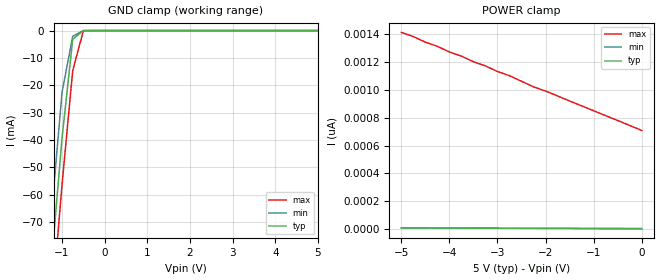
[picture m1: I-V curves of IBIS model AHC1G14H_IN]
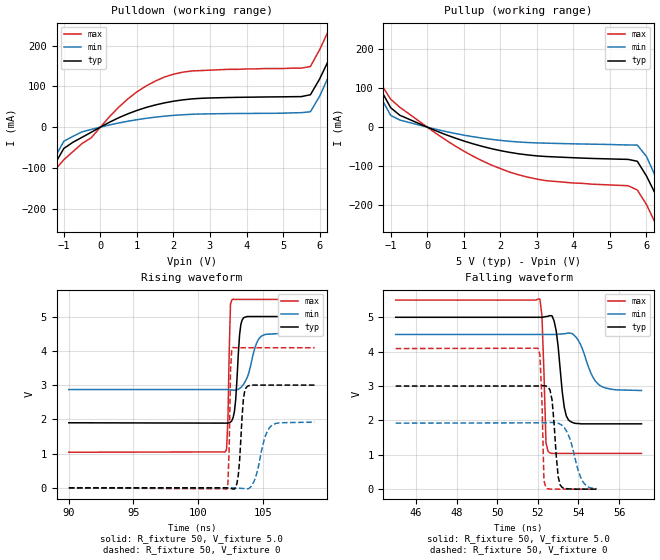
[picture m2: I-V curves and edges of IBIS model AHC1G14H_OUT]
| TEXAS INSTRUMENTS INCORPORATED
| Standard Linear and Logic Group
| IBIS Model of SN74AHC1G14H
| SINGLE SCHMITT-TRIGGER INVERTER
| CMPAK-5 5-pin (DCK) Package
[IBIS Ver]   2.1
[Comment Char]  |_char
[File name]   ul14_5c.ibs
[File Rev]   2.0
[Date]   April 17, 2000
[Source]   Data created from SPICE simulations at Hitachi,Ltd.
[Notes]   The following is an IBIS List for the AHC1G14H.
|   Please contact sllibis@ti.com with questions and
|   comments concerning SLL IBIS models.
[Disclaimer] Property of Texas Instruments Incorporated.  Unauthorized
   reproduction and/or distribution is strictly prohibited.
   This product is protected under copyright law.
   Created 2000, (C) Copyright 2000, Texas Instruments Inc.,
   All Rights Reserved.
   UNLESS THERE IS A SIGNED, WRITTEN AGREEMENT TO THE
   CONTRARY, TEXAS INSTRUMENTS () IS PROVIDING THE IBIS
   MODELS  AND WITHOUT ANY WARRANTY, EXPRESSED OR
   IMPLIED.  TI assumes no liability for:
   1) the accuracy of the IBIS models provided to your
   company;
   2) the proper functioning of these IBIS Models in your
   design or for any resulting applications; or
   3) infringement of patents, copyrights or intellectual
   property rights resulting from your use of these IBIS
   models.
   TI provides IBIS Models as a service to our customers.
   You and your company shall not distribute, sell or give
   these models to anyone else without prior written
   permission from TI.
   TI reserves the right to make changes to our products or
   to discontinue any semiconductor product or service
   without notice, and advises our customers to obtain the
   latest version of relevant information to verify, before
   placing orders, that the information being relied on is
   current.
   Please be aware that your receipt and use of the IBIS
   information provided shall serve as acceptance of these
   terms and conditions.  If you do not accept these terms,
   you should return or destroy the IBIS models and any
   other accompanying information immediately.
|   Component AHC1G14H
[Component]   AHC1G14H
[Manufacturer]   Hitachi, Ltd.
[Package]
|   typ   min   max
R_pkg   0.090   0.051   0.105
L_pkg   1.500nH   0.940nH   1.700nH
C_pkg   0.170pF   0.110pF   0.360pF
[Pin]   signal_name   model_name   R_pin   L_pin   C_pin
1   NC   NC   0.098   1.590nH   0.110pF
2   A   AHC1G14H_IN   0.051   0.940nH   0.170pF
3   GND   GND   0.092   1.590nH   0.360pF
4   Y   AHC1G14H_OUT   0.105   1.700nH   0.110pF
5   VCC   POWER   0.104   1.690nH   0.110pF
| Models and submodels in the file (2): AHC1G14H_IN (Input), AHC1G14H_OUT (Output)
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|   Model AHC1G14H_IN
[Model]   AHC1G14H_IN
Model_type  Input
Polarity   Non-Inverting
Vinl = 1.50
Vinh = 3.50
| variable   typ   min   max
C_comp   2.19pF   2.07pF   2.30pF
[Temperature Range]   25   85   -40
[Voltage Range]   5.0   4.5   5.5
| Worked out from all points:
|   GND clamp passes 1 mA (typ) near -0.58 V on its own axis
[GND Clamp]
|   Voltage   I(typ)   I(min)   I(max)
-5V       -823mA     -807mA     -840mA
-1.5V     -133mA     -115mA     -150mA
-1.25V    -85.2mA    -67.5mA    -103mA
-1V       -39.2mA    -22.5mA    -56.2mA
-750mV    -3.18mA    -2.09mA    -14.6mA
-500mV    -11.6uA    -2.99uA    -57.1uA
5V        5.34pA     5pA        708pA
[POWER Clamp]
|   Voltage   I(typ)   I(min)   I(max)
-5V       10.6pA     10pA       1.41nA
-4.75V    10.3pA     9.75pA     1.38nA
-4.5V     10pA       9.5pA      1.34nA
-4.25V    9.78pA     9.25pA     1.31nA
-4V       9.52pA     9pA        1.27nA
-3.75V    9.26pA     8.75pA     1.24nA
-3.5V     9pA        8.5pA      1.2nA
-3.25V    8.74pA     8.25pA     1.17nA
-2.75V    8.21pA     7.75pA     1.1nA
-2.25V    7.69pA     7.25pA     1.02nA
-2V       7.43pA     7pA        990pA
0V        5.34pA     5pA        708pA
|   Model AHC1G14H_OUT
[Model]   AHC1G14H_OUT
Model_type  Output
Polarity   Inverting
Vmeas = 2.5
Cref = 15pf
| variable   typ   min   max
C_comp   4.52pF   4.32pF   4.72pF
[Temperature Range]   25   85   -40
[Voltage Range]   5.0   4.5   5.5
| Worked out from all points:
|   slope of the pulldown table from 0 to 0.75 V, typ, clamps not added: 23 ohm
|   slope of the pullup table from 0 to 0.75 V, typ, clamps not added: 27.3 ohm
|   rising waveform, R_fixture 50, V_fixture 5.0: 20-80 % time 300ps typ, 710ps min, 153ps max; typ from 1.9 V to 5 V
|   falling waveform, R_fixture 50, V_fixture 5.0: 20-80 % time 320ps typ, 648ps min, 145ps max; typ from 5 V to 1.9 V
|   falling waveform, R_fixture 50, V_fixture 0: 20-80 % time 235ps typ, 547ps min, 127ps max; typ from 3 V to 0 V
|   rising waveform, R_fixture 50, V_fixture 0: 20-80 % time 302ps typ, 719ps min, 129ps max; typ from 0 V to 3 V
[Pulldown]
|   Voltage   I(typ)   I(min)   I(max)
-5V       -826mA     -810mA     -842mA
-2.25V    -282mA     -267mA     -299mA
-2V       -234mA     -219mA     -250mA
-1.25V    -91.3mA    -75.2mA    -106mA
-1V       -52.3mA    -34.7mA    -80mA
750mV     32.6mA     14.5mA     69.2mA
1.75V     59.5mA     26.9mA     123mA
5.75V     79.6mA     37.8mA     149mA
6.25V     165mA      125mA      238mA
6.75V     261mA      217mA      336mA
7V        310mA      265mA      385mA
10V       906mA      861mA      980mA
[Pullup]
|   Voltage   I(typ)   I(min)   I(max)
-5V       828mA      811mA      845mA
-2.25V    284mA      267mA      301mA
-2V       235mA      218mA      252mA
-1V       49.6mA     30.1mA     71.4mA
750mV     -27.5mA    -16mA      -47.4mA
2.25V     -64.5mA    -36.2mA    -115mA
5.75V     -87.4mA    -46mA      -161mA
6V        -125mA     -75mA      -198mA
6.25V     -172mA     -127mA     -247mA
6.75V     -269mA     -224mA     -345mA
7V        -318mA     -273mA     -395mA
10V       -917mA     -874mA     -991mA
[Ramp]
| variable   typ   min   max
dV/dt_r   1.80E+00/3.00E-10   1.15E+00/7.20E-10   2.45E+00/1.20E-10
dV/dt_f   1.86E+00/3.10E-10   9.76E-01/6.40E-10   2.68E+00/1.40E-10
R_load = 50
[Rising Waveform]
R_fixture = 50
V_fixture = 5.0
V_fixture_min = 4.5
V_fixture_max = 5.5
|   Time   V(typ)   V(min)   V(max)
90ns      1.9V       2.87V      1.04V
102.1ns   1.89V      2.87V      1.05V
102.2ns   1.89V      2.87V      1.14V
102.3ns   1.89V      2.87V      2V
102.5ns   1.92V      2.86V      5.37V
102.8ns   2.22V      2.85V      5.5V
103.2ns   4.46V      2.9V       5.5V
103.4ns   4.9V       2.97V      5.5V
104.7ns   5V         4.35V      5.5V
106.1ns   5V         4.5V       5.5V
[Falling Waveform]
R_fixture = 50
V_fixture = 5.0
V_fixture_min = 4.5
V_fixture_max = 5.5
|   Time   V(typ)   V(min)   V(max)
45ns      5V         4.5V       5.5V
52.1ns    5V         4.5V       5.53V
52.2ns    5V         4.5V       5.05V
52.4ns    5.02V      4.5V       1.34V
52.5ns    5.03V      4.5V       1.1V
52.9ns    4.61V      4.5V       1.04V
53.3ns    2.38V      4.52V      1.04V
53.5ns    2.02V      4.54V      1.04V
55ns      1.9V       3.04V      1.04V
57.1ns    1.9V       2.87V      1.04V
[Falling Waveform]
R_fixture = 50
V_fixture = 0
|   Time   V(typ)   V(min)   V(max)
45ns      3V         1.92V      4.09V
52ns      3V         1.93V      4.1V
52.1ns    3.01V      1.93V      3.92V
52.2ns    3.01V      1.93V      2.59V
52.3ns    3.01V      1.93V      250mV
52.4ns    3V         1.93V      34.6mV
52.7ns    2.59V      1.94V      456uV
53.1ns    119mV      1.89V      36uV
54.2ns    470uV      235mV      -19uV
54.9ns    -156uV     13.2mV     13uV
[Rising Waveform]
R_fixture = 50
V_fixture = 0
|   Time   V(typ)   V(min)   V(max)
90ns      0V         0V         0V
102.2ns   -401uV     646uV      -37.3mV
102.3ns   -3.51mV    798uV      122mV
102.4ns   -8.19mV    893uV      1.19V
102.5ns   -14.4mV    1.14mV     3.41V
102.6ns   -22.6mV    972uV      4.07V
103.1ns   367mV      -6.57mV    4.09V
103.7ns   2.92V      -28.2mV    4.09V
105.7ns   3V         1.83V      4.09V
109ns     3V         1.92V      4.09V
